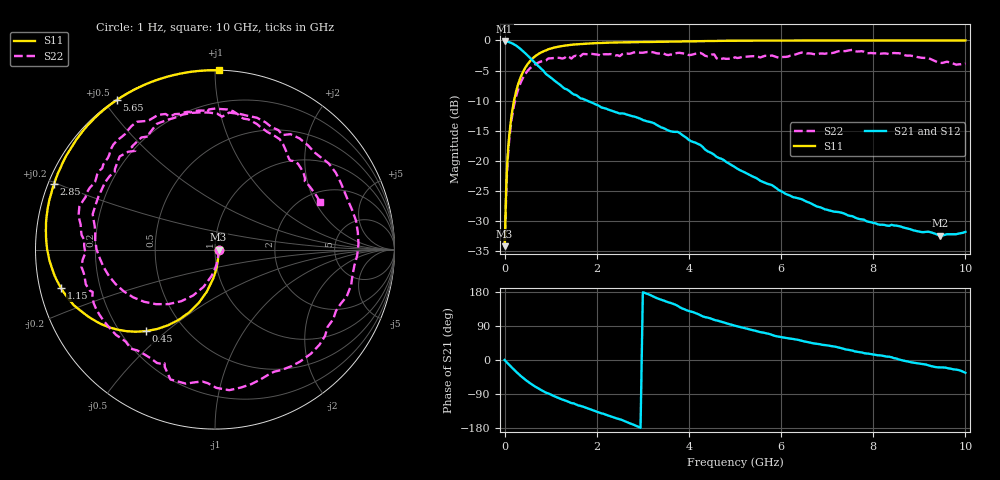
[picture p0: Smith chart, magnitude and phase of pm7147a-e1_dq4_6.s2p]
# GHz S DB R 50
! S-Parameters data
! Freq  dbS11  angS11  dbS21  angS21  dbS12  angS12  dbS22  angS22
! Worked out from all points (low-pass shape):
!   279 points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, 1 Hz to 10 GHz, reference 50 ohm
!   highest |S21| = -0.17 dB at 25.12 kHz (marker M1); lowest = -32.4 dB at 9.45 GHz (marker M2)
!   |S21| within 3 dB of the highest: start of sweep to 587.9 MHz
!   lowest |S11| = -34.2 dB at 19.95 kHz (marker M3), VSWR 1.04, Z = 52 - j0.00335 ohm
!   |S11| at or under -10 dB: start of sweep to 204.6 MHz
!   |S22| runs from -34.2 to -1.6 dB; largest |S21 - S12| = 4e-13
!   S11 on the Smith chart (normalised r, x): 1 Hz: 1.04, -0.00; 450 MHz: 0.30, -0.43; 1.15 GHz: 0.06, -0.12; 2.85 GHz: 0.02, +0.20; 5.65 GHz: 0.00, +0.54; 10 GHz: 0.00, +1.03
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1e-09  -34.17 -0.0  -0.17 -0.0  -0.17 -0.0  -34.17 -0.0
1.99526e-05  -34.17 -0.1  -0.17 -0.0  -0.17 -0.0  -34.17 -0.1
2.51189e-05  -34.17 -0.1  -0.17 -0.0  -0.17 -0.0  -34.17 -0.1
0.06309573  -19.66 -85.6  -0.22 -8.1  -0.22 -8.1  -20.37 -87.5
0.15  -12.46 -100.9  -0.43 -19.0  -0.43 -19.0  -13.22 -107.2
0.45  -4.51 -130.2  -2.14 -52.1  -2.14 -52.1  -5.55 -149.7
0.75  -2.18 -149.4  -4.37 -76.2  -4.37 -76.2  -3.61 179.9
1.15  -1.07 -166.0  -7.06 -99.2  -7.06 -99.2  -2.88 148.6
1.7  -0.56 178.8  -9.71 -123.0  -9.71 -123.0  -2.25 114.8
2.3  -0.36 166.8  -11.61 -148.7  -11.61 -148.7  -2.26 72.3
2.85  -0.28 157.9  -12.73 -173.6  -12.73 -173.6  -1.96 32.5
3.35  -0.21 150.7  -14.25 161.1  -14.25 161.1  -2.17 -10.3
3.85  -0.15 144.1  -15.67 136.2  -15.67 136.2  -2.12 -52.7
4.25  -0.11 139.1  -17.37 118.2  -17.37 118.2  -2.08 -84.2
4.55  -0.08 135.4  -19.01 105.8  -19.01 105.8  -2.33 -108.9
5.05  -0.05 129.7  -21.29 88.8  -21.29 88.8  -2.92 -134.1
5.65  -0.03 123.2  -23.63 71.1  -23.63 71.1  -2.55 -165.0
6.7  -0.01 113.1  -27.28 44.0  -27.28 44.0  -2.26 151.9
7.55  -0.01 105.8  -29.19 24.8  -29.19 24.8  -1.57 121.4
8.35  -0.01 99.6  -30.80 8.5  -30.80 8.5  -2.30 93.3
9.45  -0.00 92.0  -32.42 -19.5  -32.42 -19.5  -3.72 50.7
10  -0.00 88.6  -31.80 -33.6  -31.80 -33.6  -3.83 24.1
